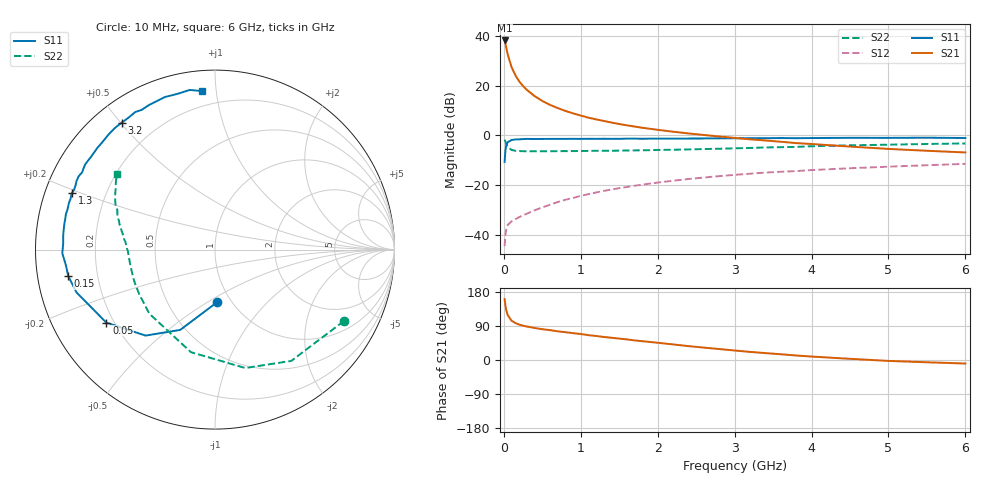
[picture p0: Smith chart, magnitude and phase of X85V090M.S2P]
! SIEMENS Small Signal Semiconductors
! BFP136W
! Si NPN RF Bipolar Junction Transistor in SOT343
! VCE = 5 V  IC = 90 mA
! Common Emitter S-Parameters:  September  1994
# GHz  S  MA  R  50
!  f  S11  S21  S12  S22
! GHz  MAG  ANG  MAG  ANG  MAG  ANG  MAG  ANG
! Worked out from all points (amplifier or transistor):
!   40 points, 10 MHz to 6 GHz, reference 50 ohm
!   highest |S21| = 38.2 dB at 10 MHz (marker M1)
!   |S21| within 3 dB of that: start of sweep to 32.08 MHz
!   unconditionally stable (mu >= 1): 565 MHz to 2.9 GHz
!   at 200 MHz: K = 0.65, MSG = 27.3 dB, |S12| = -32.9 dB
!   at 1.5 GHz: K = 1.10, MAG = 10.9 dB, |S12| = -21.2 dB
!   at 6 GHz: K = 0.96, MSG = 2.3 dB, |S12| = -11.4 dB
!   S11 on the Smith chart (normalised r, x): 10 MHz: 0.86, -0.55; 50 MHz: 0.17, -0.30; 150 MHz: 0.09, -0.09; 1.3 GHz: 0.08, +0.19; 3.2 GHz: 0.08, +0.50; 6 GHz: 0.11, +0.91
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0.01  0.2937 -87.8  81.55 160.7  0.0059 68.1  0.8212 -29.0
0.02  0.4875 -113.4  70.33 144.5  0.0096 58.9  0.7517 -55.6
0.03  0.6156 -128.9  59.76 132.9  0.0127 48.6  0.6809 -75.7
0.05  0.7294 -146.1  42.88 118.7  0.0158 39.2  0.5869 -103.2
0.1  0.8076 -162.8  23.84 103.9  0.0186 35.4  0.5112 -135.7
0.15  0.8311 -169.8  16.23 97.4  0.0206 37.6  0.4898 -149.5
0.2  0.8343 -173.6  12.21 93.4  0.0227 39.4  0.484 -156.9
0.25  0.8432 -176.6  9.846 90.5  0.0247 43.1  0.4818 -161.7
0.3  0.8511 -178.6  8.232 88.4  0.0266 45.4  0.4794 -165.0
0.4  0.8464 177.8  6.196 84.5  0.0312 49.7  0.4794 -169.2
0.5  0.8494 174.8  4.942 81.3  0.0356 52.8  0.4802 -172.2
0.6  0.8502 172.8  4.121 78.8  0.0402 55.4  0.4808 -174.0
0.7  0.8518 170.0  3.553 75.7  0.0456 57.7  0.4821 -175.4
0.9  0.8539 166.5  2.781 70.8  0.0551 59.0  0.4842 -178.0
1.1  0.8546 162.2  2.276 65.5  0.0658 60.0  0.4876 -179.7
1.3  0.8577 158.3  1.956 60.8  0.0764 60.1  0.4913 178.6
1.7  0.8622 151.6  1.508 51.7  0.0971 58.3  0.5 175.5
2.2  0.8626 143.3  1.188 41.1  0.1224 54.8  0.5144 171.9
3.2  0.878 126.3  0.835 21.4  0.1694 45.7  0.5594 163.2
4.5  0.8947 108.2  0.596 3.1  0.2185 33.6  0.6319 151.8
5.5  0.9005 99.0  0.491 -6.0  0.2513 25.8  0.6729 145.1
6  0.8863 94.7  0.454 -9.3  0.2677 21.5  0.6891 142.2
